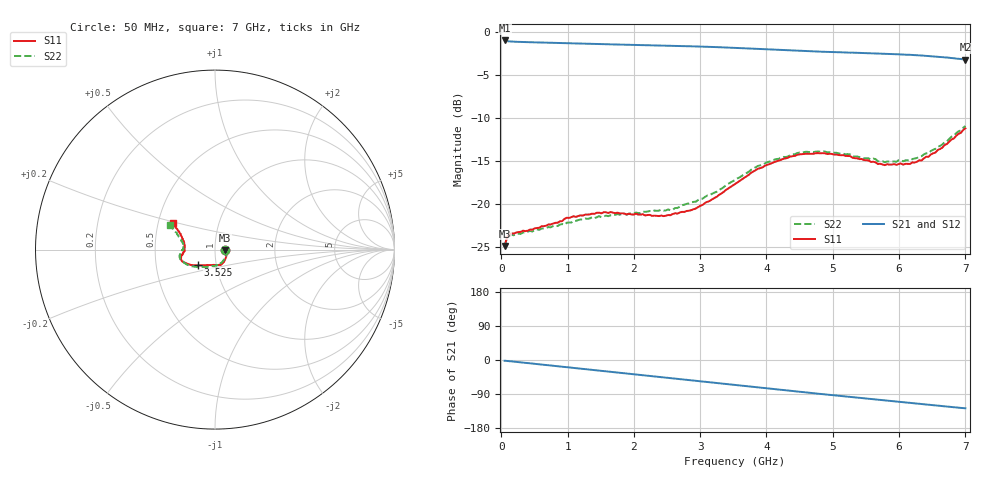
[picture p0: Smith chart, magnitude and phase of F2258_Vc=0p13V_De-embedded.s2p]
! Integrated Device Technology
! Corporate Headquarters
! 6024 Silver Creek Valley Road
! San Jose, CA 95138  USA
! Phone:  1-408-284-8200
! Toll Free:  1-800-223-1366
! Webpage:  http://www.idt.com/
! Timing and RF Division
! 515 Groton Road, Suite 102
! Westford, MA 01886-6024
! Device:  F2258
! Description: Voltage Variable RF Attenuator
! Frequency:  50.0 -  6000.00 MHz
! Package:  3x3 mm Thin QFN Plastic Package: 16 pin
! Ports:  2 RF, 2 DC
!  Pin  1  = NC
!  Pin  2  = NC
!  Pin  3  = RF2  = Port 2
!  Pin  4  = GND
!  Pin  5  = Vdd
!  Pin  6  = NC
!  Pin  7  = VCTRL
!  Pin  8  = NC
!  Pin  9  = GND
!  Pin 10  = RF1  = Port 1
!  Pin 11  = NC
!  Pin 12  = NC
!  Pin 13  = NC
!  Pin 14  = NC
!  Pin 15  = NC
!  Pin 16  = NC
! Vcntrl:  0.130 Volts
! Vdd:  +3.300 Volts
! Current:  1.076 mA
! Data:  The device was measured on a the F2258 evaluation board which has
!  individual transmission lines to the RF pins.  Data was collected
!  using a calibrated network analyzer.  The evaluation board was
!  de-embedded using a TRL calibration technique.
!  The reference plane is the edge of the package pin.
! Misc:  SN 10
!  Action Tracker AT0285
! Date Measured:  2014-12-10
! Date:  2016-01-13  MJV
! Note:
!  Integrated Device Technology supplies this data as a sample of measured
!  data at the package pin for this product.  Your particular data for this
!  product may vary.
!  Data was taken at 25 degrees C.
!  Integrated Device Technology reserves the right to change this data at anytime.
!Freq_(GHz)  S11M_(dB)  S11P_(deg)  S21M_(dB)  S21P_(deg)  S12M_(dB)  S12P_(deg)  S22M_(dB)  S22P_(deg)
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# GHz S dB R 50
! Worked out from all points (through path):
!   201 points, 50 MHz to 7 GHz, reference 50 ohm
!   highest |S21| = -0.96 dB at 50 MHz (marker M1); lowest = -3.2 dB at 7 GHz (marker M2)
!   group delay of S21, straight-line fit = 50.5 ps
!   lowest |S11| = -24.9 dB at 50 MHz (marker M3), VSWR 1.12, Z = 56 - j0.394 ohm
!   |S11| at or under -10 dB: start of sweep to end of sweep
!   |S22| runs from -24.9 to -10.9 dB; largest |S21 - S12| = 0.00044
!   S11 on the Smith chart (normalised r, x): 50 MHz: 1.12, -0.01; 3.525 GHz: 0.81, -0.14; 7 GHz: 0.60, +0.19
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0.05  -24.88 -3.5  -0.96 -1.9  -0.96 -1.9  -24.91 -3.0
0.08475  -23.91 -6.0  -1.03 -2.4  -1.03 -2.5  -23.98 -5.5
0.15425  -23.42 -9.3  -1.08 -3.6  -1.08 -3.6  -23.60 -9.4
0.71025  -22.39 -37.2  -1.22 -14.1  -1.22 -14.1  -22.69 -38.6
0.91875  -21.99 -47.0  -1.26 -18.0  -1.26 -18.0  -22.33 -50.4
0.98825  -21.60 -51.1  -1.27 -19.3  -1.27 -19.3  -22.18 -54.7
1.2315  -21.35 -59.3  -1.32 -23.8  -1.32 -23.8  -21.80 -63.8
1.6485  -20.94 -71.0  -1.41 -31.4  -1.41 -31.4  -21.31 -76.8
2.37825  -21.41 -92.4  -1.54 -44.8  -1.54 -44.8  -20.78 -94.3
2.552  -21.31 -98.4  -1.57 -48.0  -1.57 -48.0  -20.74 -99.6
2.93425  -20.53 -115.1  -1.65 -55.1  -1.65 -55.1  -19.73 -113.0
3.525  -17.70 -137.8  -1.82 -66.2  -1.82 -66.2  -17.21 -135.6
4.0115  -15.42 -151.4  -2.00 -75.2  -2.00 -75.2  -15.12 -151.0
4.46325  -14.28 -159.8  -2.16 -83.4  -2.16 -83.4  -14.07 -162.1
4.7065  -14.15 -163.1  -2.23 -87.7  -2.23 -87.7  -13.96 -166.3
5.2625  -14.42 -170.0  -2.38 -97.4  -2.38 -97.3  -14.21 -174.3
5.6795  -15.35 -176.8  -2.47 -104.6  -2.47 -104.6  -15.03 -179.7
5.85325  -15.41 179.0  -2.52 -107.8  -2.52 -107.8  -15.06 175.7
6.166  -15.34 171.2  -2.63 -113.4  -2.63 -113.3  -14.97 169.8
6.33975  -14.93 164.9  -2.71 -116.5  -2.71 -116.5  -14.43 165.4
6.722  -13.01 153.3  -2.94 -123.1  -2.95 -123.1  -12.72 156.4
7  -11.19 147.9  -3.19 -127.4  -3.19 -127.4  -10.92 151.5
